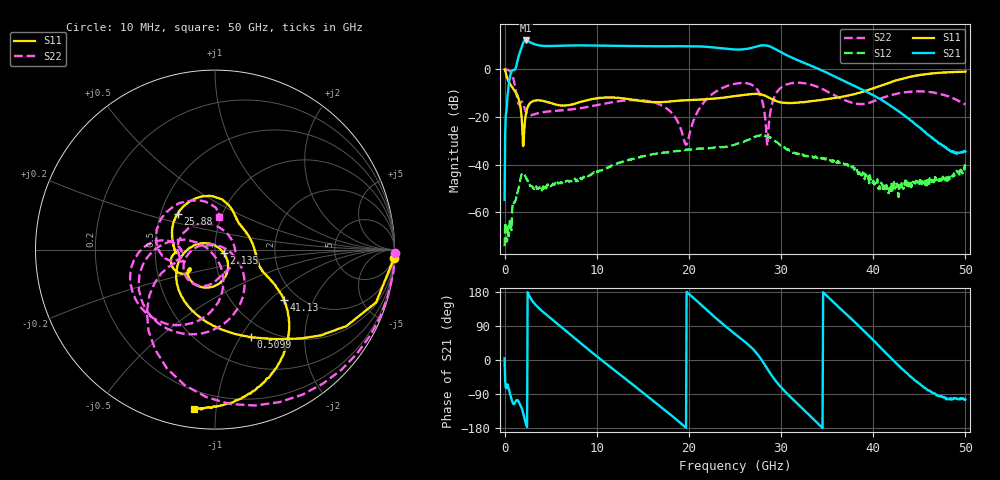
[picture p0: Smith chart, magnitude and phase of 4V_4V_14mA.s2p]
! MARKI MICROWAVE INC.
! Date:  1/07/2020
! Model Number:  APM-6849CH
! Description:  2-port Small Signal S-parameter data for APM-6849CH
! Frequency Range:  10 MHz to 50 GHz
! Port Configuration:  PORT 1: Input
!  PORT 2: Output
! Bias Condition: Vc = +4V, Vb = +4V
! APM-6849CH s2p files are only valid for small signal conditions (below -5 dBm input power)
!S2P File: Measurements: Mag<S11> Ang<S11>, Mag<S21> Ang<S21>, Mag<S12> Ang<S12>, Mag<S22> Ang<S22>!row 1
# Hz S  dB  R 50
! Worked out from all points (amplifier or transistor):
!   801 points, 10 MHz to 50 GHz, reference 50 ohm
!   highest |S21| = 12.1 dB at 2.322 GHz (marker M1)
!   |S21| within 3 dB of that: 1.84 GHz to 22.83 GHz (20.99 GHz wide, 170 % of centre)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
!   unconditionally stable (mu >= 1): 103.3 MHz to end of sweep
!   at 8.321 GHz: K = 29.64, MAG = 10.4 dB, |S12| = -46.1 dB
!   at 25 GHz: K = 5.11, MAG = 9.9 dB, |S12| = -31.6 dB
!   at 50 GHz: K = 528.85, MAG = -27.2 dB, |S12| = -40.5 dB
!   S11 on the Smith chart (normalised r, x): 10 MHz: 1, -43; 509.9 MHz: 0.82, -1.12; 2.135 GHz: 1.10, -0.04; 25.88 GHz: 0.61, +0.27; 41.13 GHz: 1.69, -1.24; 50 GHz: 0.09, -0.87
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1e7  -0.01 -2.7  -54.82 4.4  -74.31 -79.7  0.04 -1.1
5.099e8  -5.55 -67.5  -5.07 -80.2  -68.50 6.5  -0.50 -59.0
1.5097e9  -12.10 -150.2  5.13 -108.9  -50.35 -79.7  -14.50 -159.8
2.134575e9  -25.83 -18.7  11.83 -151.1  -44.19 -153.2  -15.92 114.8
2.322038e9  -18.72 -50.9  12.14 -167.8  -45.38 -170.1  -17.94 80.1
3.071888e9  -13.39 -99.4  10.85 154.2  -49.58 170.2  -19.09 1.4
4.634075e9  -13.73 -137.3  9.81 117.7  -48.59 163.4  -17.75 -45.1
8.383325e9  -13.56 -140.5  10.07 41.8  -46.21 126.5  -16.23 -80.3
1.182014e10  -11.85 -163.5  9.89 -24.9  -40.08 94.0  -13.75 -102.8
1.438212e10  -13.07 -175.3  9.77 -73.8  -37.17 57.4  -12.91 -127.7
1.669416e10  -13.81 -174.8  9.71 -118.4  -35.29 21.3  -14.53 -157.2
2.038092e10  -12.86 178.0  9.70 166.4  -33.68 -38.0  -22.92 -3.0
2.269296e10  -12.29 167.4  9.20 115.7  -33.05 -81.2  -9.97 -61.9
2.5005e10  -11.23 148.1  8.35 68.6  -31.61 -124.6  -6.08 -108.6
2.587982e10  -10.80 135.9  8.41 51.9  -30.50 -146.8  -5.72 -128.1
2.80044e10  -10.76 88.6  10.10 -4.1  -27.86 138.3  -13.98 164.5
2.937912e10  -13.19 59.1  8.53 -53.9  -30.08 79.4  -10.67 -86.3
3.112878e10  -14.14 35.5  5.00 -100.1  -34.38 39.0  -5.83 -130.8
3.337832e10  -13.36 5.4  1.29 -152.7  -36.58 -0.7  -6.59 -169.8
4.112678e10  -6.41 -36.2  -13.39 24.8  -51.39 89.1  -11.86 -166.2
4.168916e10  -5.67 -39.6  -14.81 10.8  -52.01 97.5  -11.11 -169.9
5e10  -0.94 -97.6  -34.50 -104.6  -40.52 -79.6  -14.86 82.8
